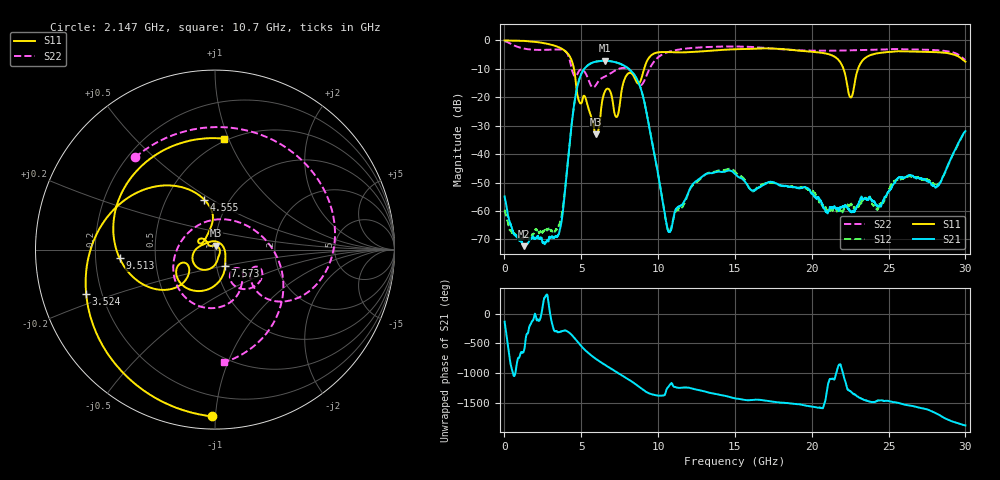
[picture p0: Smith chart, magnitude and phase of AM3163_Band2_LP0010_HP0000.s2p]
!Agilent Technologies,E8364B,MY43040894,A.07.50.67
!Agilent E8364B: A.07.50.67
!Date: Thursday, August 20, 2020 12:04:59
!Correction: S11(Full 2 Port(1,2))
!S21(Full 2 Port(1,2))
!S12(Full 2 Port(1,2))
!S22(Full 2 Port(1,2))
!S2P File: Measurements: S11, S21, S12, S22:
# Hz S  dB  R 50
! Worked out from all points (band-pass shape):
!   3201 points, 10 MHz to 30 GHz, reference 50 ohm
!   highest |S21| = -7.17 dB at 6.514 GHz (marker M1); lowest = -72.4 dB at 1.275 GHz (marker M2)
!   |S21| within 3 dB of the highest: 5.179 GHz to 8.129 GHz (2.95 GHz wide, 44.3 % of centre)
!   lowest |S11| = -33.1 dB at 5.952 GHz (marker M3), VSWR 1.05, Z = 50.4 + j2.19 ohm
!   |S11| at or under -10 dB: 4.524 GHz to 9.091 GHz (4.567 GHz wide, 67.1 % of centre); 22.07 GHz to 23.01 GHz (946.7 MHz wide, 4.2 % of centre)
!   |S22| runs from -16.6 to -0.3 dB; largest |S21 - S12| = 0.0033
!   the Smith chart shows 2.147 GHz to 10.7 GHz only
!   S11 on the Smith chart (normalised r, x): 2.147 GHz: 0.07, -0.98; 3.524 GHz: 0.14, -0.16; 4.555 GHz: 0.77, +0.46; 7.573 GHz: 1.10, -0.20; 9.513 GHz: 0.30, -0.04; 10.7 GHz: 0.48, +0.96
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1e7  -0.04 -2.8  -54.89 -134.9  -59.51 -100.8  -0.28 -11.4
5.535688e8  -0.06 -22.7  -67.07 77.4  -67.80 -152.9  -1.61 -84.6
1.275203e9  -0.19 -53.0  -72.36 104.0  -69.84 25.1  -2.89 -161.6
2.146788e9  -0.63 -90.9  -68.76 -104.6  -66.65 121.4  -3.36 131.0
3.524453e9  -2.40 -161.2  -68.34 49.4  -65.24 53.4  -3.17 33.7
4.555359e9  -10.93 102.0  -21.86 -49.4  -21.87 -49.8  -12.53 -33.9
5.014581e9  -22.03 150.4  -11.67 169.1  -11.67 168.9  -10.28 -36.9
5.951769e9  -33.08 78.9  -7.48 -39.9  -7.49 -40.0  -15.70 -38.8
6.514081e9  -18.24 -113.3  -7.17 -136.2  -7.17 -136.4  -12.77 -48.2
7.573103e9  -19.45 -57.6  -8.31 57.1  -8.36 57.1  -9.80 -87.6
8.322853e9  -11.88 -148.0  -11.21 -66.7  -11.21 -66.6  -11.54 -150.7
9.513081e9  -5.46 -174.8  -33.20 91.8  -33.00 91.2  -9.30 -5.4
1.000979e10  -4.21 140.2  -47.35 62.5  -47.34 61.8  -5.93 -46.7
1.070331e10  -4.15 85.6  -67.40 -135.6  -66.96 144.7  -4.01 -85.4
1.221218e10  -4.11 -15.1  -50.91 -176.5  -51.20 -176.0  -2.68 -142.8
1.5005e10  -3.12 -144.1  -47.00 17.7  -46.13 17.8  -2.14 126.7
1.768536e10  -2.92 93.9  -50.28 -46.0  -50.35 -47.9  -2.99 28.0
2.000958e10  -4.01 -30.5  -53.89 -121.3  -52.84 -124.7  -3.62 -52.5
2.253999e10  -20.08 -105.1  -60.15 134.1  -57.83 -171.4  -3.51 -123.4
2.500479e10  -4.09 -151.8  -53.03 -26.4  -52.61 -29.6  -3.20 176.4
2.819123e10  -4.17 107.7  -51.32 115.7  -50.75 113.8  -3.49 91.3
3e10  -7.48 38.4  -31.90 -77.9  -32.13 -80.2  -6.98 35.8
